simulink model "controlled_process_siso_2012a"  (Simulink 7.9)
settings: Solver=ode3  StartTime=0.0  StopTime=simopt.Tf  FixedStep=simopt.h  RelTol=1e-3
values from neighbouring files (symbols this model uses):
  simopt = []    [setParams.m]
libraries: cstblocks x1

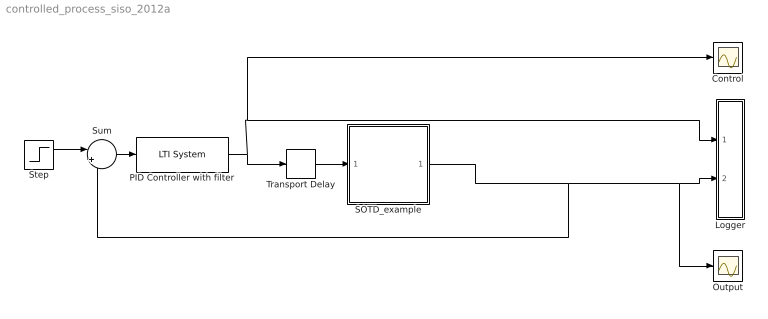
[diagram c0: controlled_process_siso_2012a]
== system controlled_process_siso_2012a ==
  Control : Scope
  Logger : Subsystem
  Output : Scope
  PID Controller with filter : cstblocks/LTI System  sys=FC  IC=[]
  SOTD_example : Subsystem
  Step : Step  Time=100  Before=2  After=4  SampleTime=simopt.h
  Sum : Sum  Inputs=|+-
  Transport Delay : TransportDelay  DelayTime=0
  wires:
  Step/1 -> Sum/1
  PID Controller with filter/1 -> Control/1, Logger/1(u1), Transport Delay/1
  Sum/1 -> PID Controller with filter/1
  SOTD_example/1(y) -> Logger/2(y1), Output/1, Sum/2
  Transport Delay/1 -> SOTD_example/1(u)

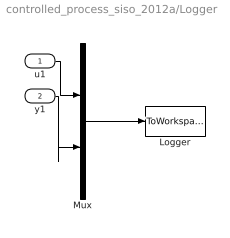
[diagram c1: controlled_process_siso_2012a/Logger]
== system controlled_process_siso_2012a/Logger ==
  u1 : Inport  SampleTime=simopt.h
  y1 : Inport  Port=2  SampleTime=simopt.h
  Logger : ToWorkspace  VariableName=simout  SampleTime=simopt.h  SaveFormat=Structure With Time
  Mux : Mux  Inputs=2
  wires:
  Mux/1 -> Logger/1
  u1/1 -> Mux/1
  y1/1 -> Mux/2

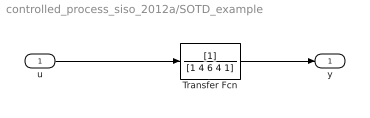
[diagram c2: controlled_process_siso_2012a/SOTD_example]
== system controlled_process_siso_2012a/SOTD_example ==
  u : Inport  SampleTime=simopt.h
  Transfer Fcn : TransferFcn  Denominator=[1 4 6 4 1]
  y : Outport  SampleTime=simopt.h
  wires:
  u/1 -> Transfer Fcn/1
  Transfer Fcn/1 -> y/1
